| TEXAS INSTRUMENTS INCORPORATED
| Standard Linear and Logic Group
| IBIS Model of LVTH16245A
| 16-Bit Bus Transceiver with 3-State Outputs
| This file contains package information for the following:
|  SSOP 48-pin (DL) package as [Component] LVTH16245A_DL
|  TSSOP 48-pin (DGG) package as [Component] LVTH16245A_DGG
|  TVSOP 48-pin (DGV) package as [Component] LVTH16245A_DGV
|  jrBGA 48-pin (GQL) package as [Component] LVTH16245A_GQL
| This device can be powered at the following Vccs:
|  3.3 volt Vcc
|  2.7 volt Vcc
| This file provides unique models under the [Model Selector] for each Vcc.
| For operation at a specific Vcc, select the appropriate model after each
| [Model Selector] keyword.
[IBIS Ver]   3.2
[Comment char]  |_char
[File Name]   sn54lvth16245awd.ibs
[File Rev]   1.1 | g_die
[Date]   October 15, 2008
[Source]   Data created from TI-SPICE simulations at TI-SLL.
[Notes]   The following is an IBIS list for the LVTH16245A.
   Please contact sllibis@ti.com with questions and
   comments concerning SLL IBIS models.
   - FILE REV HISTORY
   - 1.1 Release IBIS file on 10/15/08
   - Power-clamp data has been deleted since there is no
   power-clamp diode in the device.
   - Due to presence of bus hold at input, GND-clamp curves
   have non-monotonic warnings.
   - Due to the fact that the device is 5-V input/output
   tolerant, the pullup and pulldown data has some
   non-monotonic warnings.
|08/13/2013  - Updated with ceramic 48WD parasitics.  WVB
[Disclaimer] Property of Texas Instruments Incorporated.  Unauthorized
   reproduction and/or distribution is strictly prohibited.
   This product is protected under copyright law.
   Created  2008, (C) Copyright  2008, Texas Instruments
   Incorporated, All Rights Reserved
   UNLESS THERE IS A SIGNED, WRITTEN AGREEMENT TO THE
   CONTRARY, TEXAS INSTRUMENTS (TI) IS PROVIDING THE IBIS
   MODELS  AND WITHOUT ANY WARRANTY, EXPRESSED OR
   IMPLIED.  TI assumes no liability for:
   1) the accuracy of the IBIS models provided to your
   company;
   2) the proper functioning of these IBIS Models in your
   design or for any resulting applications; or
   3) infringement of patents, copyrights or intellectual
   property rights resulting from your use of these IBIS
   models.
   TI provides IBIS Models as a service to our customers.
   You and your company shall not distribute, sell or give
   these models to anyone else without prior written
   permission from TI.
   TI reserves the right to make changes to our products or
   to discontinue any semiconductor product or service
   without notice, and advises our customers to obtain the
   latest version of relevant information to verify, before
   placing orders, that the information being relied on is
   current.
   Please be aware that your receipt and use of the IBIS
   information provided shall serve as acceptance of these
   terms and conditions.  If you do not accept these terms,
   you should return or destroy the IBIS models and any
   other accompanying information immediately.
|   48-pin ceramic (WD) packageP
[Component]   LVTH16245A_DL
[Manufacturer]   Texas Instruments, Inc.
[Package]
|   typ   min   max
R_pkg   0.161   0.116   0.231
L_pkg   6.816e-9   4.867e-9   10.108e-9
C_pkg   2.468e-12   1.62e-12   3.698e-12
[Pin]   signal_name   model_name   R_pin   L_pin   C_pin
1   S1DIR   LVTH16245E_IN   0.231   10.108e-9   3.220e-12
2   S1B1   LVTH16245E_IO   0.224   9.570e-9   3.698e-12
3   S1B2   LVTH16245E_IO   0.202   8.681e-9   3.350e-12
4   GND   GND   0.185   7.877e-9   2.960e-12
5   S1B3   LVTH16245E_IO   0.170   7.118e-9   2.404e-12
6   S1B4   LVTH16245E_IO   0.155   6.481e-9   2.131e-12
7   VCC   POWER   0.138   5.760e-9   2.150e-12
8   S1B5   LVTH16245E_IO   0.135   5.641e-9   2.103e-12
9   S1B6   LVTH16245E_IO   0.134   5.593e-9   2.070e-12
10   GND   GND   0.120   5.070e-9   1.812e-12
11   S1B7   LVTH16245E_IO   0.119   5.022e-9   1.793e-12
12   S1B8   LVTH16245E_IO   0.116   4.868e-9   1.651e-12
13   S2B1   LVTH16245E_IO   0.116   4.867e-9   1.658e-12
14   S2B2   LVTH16245E_IO   0.119   5.024e-9   1.805e-12
15   GND   GND   0.121   5.074e-9   1.825e-12
16   S2B3   LVTH16245E_IO   0.134   5.595e-9   2.105e-12
17   S2B4   LVTH16245E_IO   0.136   5.644e-9   2.144e-12
18   VCC   POWER   0.139   5.763e-9   2.197e-12
19   S2B5   LVTH16245E_IO   0.155   6.483e-9   2.152e-12
20   S2B6   LVTH16245E_IO   0.157   6.535e-9   2.172e-12
21   GND   GND   0.164   6.944e-9   2.459e-12
22   S2B7   LVTH16245E_IO   0.174   7.397e-9   2.657e-12
23   S2B8   LVTH16245E_IO   0.189   7.964e-9   2.834e-12
24   S2DIR   LVTH16245E_IN   0.188   8.149e-9   2.455e-12
25   S2NOE   LVTH16245E_IN   0.188   8.148e-9   2.455e-12
26   S2A8   LVTH16245E_IO   0.189   7.963e-9   2.834e-12
27   S2A7   LVTH16245E_IO   0.174   7.396e-9   2.658e-12
28   GND   GND   0.164   6.943e-9   2.461e-12
29   S2A6   LVTH16245E_IO   0.157   6.535e-9   2.174e-12
30   S2A5   LVTH16245E_IO   0.168   7.064e-9   2.384e-12
31   VCC   POWER   0.159   6.694e-9   2.687e-12
32   S2A4   LVTH16245E_IO   0.163   6.925e-9   2.828e-12
33   S2A3   LVTH16245E_IO   0.169   7.198e-9   2.967e-12
34   GND   GND   0.163   7.027e-9   2.887e-12
35   S2A2   LVTH16245E_IO   0.162   6.977e-9   2.868e-12
36   S2A1   LVTH16245E_IO   0.167   7.207e-9   2.815e-12
37   S1A8   LVTH16245E_IO   0.149   6.371e-9   2.557e-12
38   S1A7   LVTH16245E_IO   0.139   5.942e-9   2.312e-12
39   GND   GND   0.149   6.375e-9   2.428e-12
40   S1A6   LVTH16245E_IO   0.135   5.649e-9   2.135e-12
41   S1A5   LVTH16245E_IO   0.137   5.708e-9   2.174e-12
42   VCC   POWER   0.129   5.341e-9   1.804e-12
43   S1A4   LVTH16245E_IO   0.124   5.115e-9   1.620e-12
44   S1A3   LVTH16245E_IO   0.170   7.117e-9   2.402e-12
45   GND   GND   0.185   7.876e-9   2.956e-12
46   S1A2   LVTH16245E_IO   0.202   8.680e-9   3.347e-12
47   S1A1   LVTH16245E_IO   0.224   9.570e-9   3.696e-12
48   S1NOE   LVTH16245E_IN   0.231   10.108e-9   3.219e-12
| Component LVTH16245A_DGG 48-PIN TSSOP
[Component]   LVTH16245A_DGG
[Manufacturer]   Texas Instruments, Inc.
[Package]
|   typ   min   max
R_pkg   4.400e-02   3.800e-02   5.100e-02
L_pkg   3.019e-09   2.486e-09   4.099e-09
C_pkg   5.070e-13   3.340e-13   8.090e-13
[Pin]   signal_name   model_name   R_pin   L_pin   C_pin
1   S1DIR   LVTH16245E_IN   4.100e-02   4.017e-09   7.590e-13
2   S1B1   LVTH16245E_IO   4.200e-02   3.737e-09   7.920e-13
3   S1B2   LVTH16245E_IO   4.200e-02   3.480e-09   6.610e-13
4   GND   GND   3.800e-02   3.131e-09   5.750e-13
5   S1B3   LVTH16245E_IO   4.700e-02   3.122e-09   5.660e-13
6   S1B4   LVTH16245E_IO   4.300e-02   2.948e-09   5.040e-13
7   VCC   POWER   4.500e-02   2.845e-09   3.970e-13
8   S1B5   LVTH16245E_IO   4.900e-02   2.835e-09   3.940e-13
9   S1B6   LVTH16245E_IO   4.800e-02   2.715e-09   3.780e-13
10   GND   GND   5.000e-02   2.664e-09   3.630e-13
11   S1B7   LVTH16245E_IO   5.000e-02   2.585e-09   3.480e-13
12   S1B8   LVTH16245E_IO   4.900e-02   2.550e-09   3.370e-13
13   S2B1   LVTH16245E_IO   4.900e-02   2.541e-09   3.360e-13
14   S2B2   LVTH16245E_IO   5.000e-02   2.574e-09   3.480e-13
15   GND   GND   4.900e-02   2.618e-09   3.590e-13
16   S2B3   LVTH16245E_IO   4.600e-02   2.671e-09   3.750e-13
17   S2B4   LVTH16245E_IO   4.500e-02   2.754e-09   3.890e-13
18   VCC   POWER   4.400e-02   2.823e-09   4.500e-13
19   S2B5   LVTH16245E_IO   4.200e-02   2.968e-09   5.030e-13
20   S2B6   LVTH16245E_IO   5.100e-02   3.108e-09   5.350e-13
21   GND   GND   4.200e-02   3.175e-09   5.870e-13
22   S2B7   LVTH16245E_IO   4.100e-02   3.449e-09   6.780e-13
23   S2B8   LVTH16245E_IO   4.400e-02   3.766e-09   8.040e-13
24   S2DIR   LVTH16245E_IN   4.300e-02   4.065e-09   7.610e-13
25   S2NOE   LVTH16245E_IN   4.100e-02   3.994e-09   7.570e-13
26   S2A8   LVTH16245E_IO   3.900e-02   3.649e-09   7.890e-13
27   S2A7   LVTH16245E_IO   3.800e-02   3.362e-09   6.600e-13
28   GND   GND   3.800e-02   3.082e-09   5.740e-13
29   S2A6   LVTH16245E_IO   4.400e-02   2.990e-09   5.220e-13
30   S2A5   LVTH16245E_IO   4.100e-02   2.917e-09   4.950e-13
31   VCC   POWER   4.300e-02   2.820e-09   4.480e-13
32   S2A4   LVTH16245E_IO   4.300e-02   2.699e-09   3.850e-13
33   S2A3   LVTH16245E_IO   4.500e-02   2.628e-09   3.720e-13
34   GND   GND   4.600e-02   2.556e-09   3.560e-13
35   S2A2   LVTH16245E_IO   4.600e-02   2.495e-09   3.440e-13
36   S2A1   LVTH16245E_IO   4.700e-02   2.487e-09   3.340e-13
37   S1A8   LVTH16245E_IO   4.700e-02   2.490e-09   3.350e-13
38   S1A7   LVTH16245E_IO   4.600e-02   2.486e-09   3.430e-13
39   GND   GND   4.500e-02   2.566e-09   3.560e-13
40   S1A6   LVTH16245E_IO   4.400e-02   2.639e-09   3.740e-13
41   S1A5   LVTH16245E_IO   4.300e-02   2.701e-09   3.860e-13
42   VCC   POWER   4.300e-02   2.817e-09   4.500e-13
43   S1A4   LVTH16245E_IO   4.100e-02   2.935e-09   5.010e-13
44   S1A3   LVTH16245E_IO   4.700e-02   3.035e-09   5.290e-13
45   GND   GND   4.300e-02   3.171e-09   5.890e-13
46   S1A2   LVTH16245E_IO   4.000e-02   3.415e-09   6.820e-13
47   S1A1   LVTH16245E_IO   4.300e-02   3.741e-09   8.090e-13
48   S1NOE   LVTH16245E_IN   4.400e-02   4.099e-09   7.640e-13
| Component LVTH16245A_DGV 48-PIN TVSOP
[Component]   LVTH16245A_DGV
[Manufacturer]   Texas Instruments, Inc.
[Package]
|   typ   min   max
R_pkg   1.370e-01   1.010e-01   1.720e-01
L_pkg   3.632e-09   2.739e-09   5.243e-09
C_pkg   5.430e-13   4.100e-13   7.930e-13
[Pin]   signal_name   model_name   R_pin   L_pin   C_pin
1   S1DIR   LVTH16245E_IN   1.680e-01   5.238e-09   7.750e-13
2   S1B1   LVTH16245E_IO   1.660e-01   4.546e-09   6.740e-13
3   S1B2   LVTH16245E_IO   1.700e-01   4.356e-09   6.200e-13
4   GND   GND   1.720e-01   4.192e-09   5.310e-13
5   S1B3   LVTH16245E_IO   1.570e-01   3.821e-09   5.020e-13
6   S1B4   LVTH16245E_IO   1.430e-01   3.623e-09   5.600e-13
7   VCC   POWER   1.300e-01   3.292e-09   5.060e-13
8   S1B5   LVTH16245E_IO   1.190e-01   3.090e-09   4.520e-13
9   S1B6   LVTH16245E_IO   1.110e-01   2.927e-09   4.440e-13
10   GND   GND   1.050e-01   2.807e-09   4.350e-13
11   S1B7   LVTH16245E_IO   1.010e-01   2.739e-09   4.260e-13
12   S1B8   LVTH16245E_IO   1.020e-01   2.949e-09   5.040e-13
13   S2B1   LVTH16245E_IO   1.020e-01   2.960e-09   4.800e-13
14   S2B2   LVTH16245E_IO   1.010e-01   2.747e-09   4.100e-13
15   GND   GND   1.050e-01   2.809e-09   4.350e-13
16   S2B3   LVTH16245E_IO   1.110e-01   2.928e-09   4.440e-13
17   S2B4   LVTH16245E_IO   1.190e-01   3.090e-09   4.520e-13
18   VCC   POWER   1.300e-01   3.293e-09   5.120e-13
19   S2B5   LVTH16245E_IO   1.430e-01   3.622e-09   5.750e-13
20   S2B6   LVTH16245E_IO   1.570e-01   3.818e-09   5.200e-13
21   GND   GND   1.720e-01   4.186e-09   5.560e-13
22   S2B7   LVTH16245E_IO   1.700e-01   4.354e-09   6.430e-13
23   S2B8   LVTH16245E_IO   1.660e-01   4.544e-09   6.970e-13
24   S2DIR   LVTH16245E_IN   1.680e-01   5.240e-09   7.930e-13
25   S2NOE   LVTH16245E_IN   1.680e-01   5.243e-09   7.900e-13
26   S2A8   LVTH16245E_IO   1.660e-01   4.544e-09   6.940e-13
27   S2A7   LVTH16245E_IO   1.700e-01   4.351e-09   6.460e-13
28   GND   GND   1.720e-01   4.185e-09   5.630e-13
29   S2A6   LVTH16245E_IO   1.570e-01   3.817e-09   5.270e-13
30   S2A5   LVTH16245E_IO   1.430e-01   3.622e-09   5.790e-13
31   VCC   POWER   1.300e-01   3.293e-09   5.140e-13
32   S2A4   LVTH16245E_IO   1.190e-01   3.091e-09   4.560e-13
33   S2A3   LVTH16245E_IO   1.110e-01   2.928e-09   4.480e-13
34   GND   GND   1.050e-01   2.810e-09   4.380e-13
35   S2A2   LVTH16245E_IO   1.010e-01   2.748e-09   4.140e-13
36   S2A1   LVTH16245E_IO   1.020e-01   2.959e-09   4.830e-13
37   S1A8   LVTH16245E_IO   1.020e-01   2.949e-09   5.080e-13
38   S1A7   LVTH16245E_IO   1.010e-01   2.739e-09   4.300e-13
39   GND   GND   1.050e-01   2.806e-09   4.380e-13
40   S1A6   LVTH16245E_IO   1.110e-01   2.927e-09   4.480e-13
41   S1A5   LVTH16245E_IO   1.190e-01   3.091e-09   4.560e-13
42   VCC   POWER   1.300e-01   3.292e-09   5.110e-13
43   S1A4   LVTH16245E_IO   1.430e-01   3.623e-09   5.700e-13
44   S1A3   LVTH16245E_IO   1.570e-01   3.820e-09   5.150e-13
45   GND   GND   1.720e-01   4.189e-09   5.500e-13
46   S1A2   LVTH16245E_IO   1.700e-01   4.356e-09   6.370e-13
47   S1A1   LVTH16245E_IO   1.660e-01   4.547e-09   6.930e-13
48   S1NOE   LVTH16245E_IN   1.680e-01   5.233e-09   7.900e-13
| Component LVTH16245E_GQL 48-PIN JRBGA
[Component]   LVTH16245A_GQL
[Manufacturer]   Texas Instruments, Inc.
[Package]
|   typ   min   max
R_pkg   7.900e-02   4.500e-02   9.400e-02
L_pkg   2.264e-09   1.398e-09   2.722e-09
C_pkg   3.060e-13   1.170e-13   4.040e-13
[Pin]   signal_name   model_name   R_pin   L_pin   C_pin
A1   1DIR   LVTH16245E_DIR   5.100e-02   1.531e-09   2.100e-13
B2   1B1   LVTH16245E_IO   7.300e-02   2.572e-09   3.120e-13
B1   1B2   LVTH16245E_IO   7.100e-02   1.835e-09   2.320e-13
B3   GND   GND   9.400e-02   2.717e-09   3.830e-13
C2   1B3   LVTH16245E_IO   8.900e-02   2.534e-09   3.500e-13
C1   1B4   LVTH16245E_IO   7.100e-02   1.831e-09   2.310e-13
C3   VCC   POWER   9.400e-02   2.722e-09   3.920e-13
D2   1B5   LVTH16245E_IO   9.000e-02   2.551e-09   3.520e-13
D1   1B6   LVTH16245E_IO   7.200e-02   1.846e-09   2.440e-13
D3   GND   GND   9.400e-02   2.719e-09   4.030e-13
E2   1B7   LVTH16245E_IO   8.900e-02   2.541e-09   3.510e-13
E1   1B8   LVTH16245E_IO   7.200e-02   1.850e-09   2.270e-13
F1   2B1   LVTH16245E_IO   7.200e-02   1.850e-09   2.270e-13
F2   2B2   LVTH16245E_IO   8.900e-02   2.541e-09   3.510e-13
G3   GND   GND   9.400e-02   2.718e-09   4.040e-13
G1   2B3   LVTH16245E_IO   7.200e-02   1.847e-09   2.440e-13
G2   2B4   LVTH16245E_IO   9.000e-02   2.551e-09   3.520e-13
H3   VCC   POWER   9.400e-02   2.721e-09   3.920e-13
H1   2B5   LVTH16245E_IO   7.000e-02   1.830e-09   2.310e-13
H2   2B6   LVTH16245E_IO   8.800e-02   2.524e-09   3.500e-13
J3   GND   GND   9.300e-02   2.709e-09   3.820e-13
J1   2B7   LVTH16245E_IO   7.100e-02   1.851e-09   2.330e-13
J2   2B8   LVTH16245E_IO   5.600e-02   2.605e-09   3.900e-13
K1   2DIR   LVTH16245E_DIR   4.500e-02   1.398e-09   1.170e-13
K6   2NOE   LVTH16245E_NOE   4.500e-02   1.512e-09   1.930e-13
J5   2A8   LVTH16245E_IO   5.500e-02   2.492e-09   3.130e-13
J6   2A7   LVTH16245E_IO   7.000e-02   1.821e-09   2.300e-13
J4   GND   GND   9.300e-02   2.703e-09   3.820e-13
H5   2A6   LVTH16245E_IO   8.900e-02   2.529e-09   3.500e-13
H6   2A5   LVTH16245E_IO   7.100e-02   1.826e-09   2.300e-13
H4   VCC   POWER   9.400e-02   2.722e-09   3.910e-13
G5   2A4   LVTH16245E_IO   9.000e-02   2.551e-09   3.520e-13
G6   2A3   LVTH16245E_IO   7.200e-02   1.846e-09   2.440e-13
G4   GND   GND   9.400e-02   2.719e-09   4.040e-13
F5   2A2   LVTH16245E_IO   8.800e-02   2.510e-09   3.490e-13
F6   2A1   LVTH16245E_IO   7.200e-02   1.850e-09   2.270e-13
E6   1A8   LVTH16245E_IO   7.100e-02   1.850e-09   2.270e-13
E5   1A7   LVTH16245E_IO   8.900e-02   2.529e-09   3.500e-13
D4   GND   GND   9.400e-02   2.719e-09   4.030e-13
D6   1A6   LVTH16245E_IO   7.200e-02   1.847e-09   2.430e-13
D5   1A5   LVTH16245E_IO   8.900e-02   2.550e-09   3.520e-13
C4   VCC   POWER   9.400e-02   2.722e-09   3.910e-13
C6   1A4   LVTH16245E_IO   7.100e-02   1.827e-09   2.300e-13
C5   1A3   LVTH16245E_IO   8.900e-02   2.539e-09   3.500e-13
B4   GND   GND   9.300e-02   2.705e-09   3.820e-13
B6   1A2   LVTH16245E_IO   7.100e-02   1.831e-09   2.270e-13
B5   1A1   LVTH16245E_IO   7.300e-02   2.685e-09   3.800e-13
A6   1NOE   LVTH16245E_NOE   5.100e-02   1.417e-09   1.330e-13
| Model LVTH16245E_NOE
[Model Selector]   LVTH16245E_NOE
LVTH16245E_NOE_33   3.3 volt Vcc
LVTH16245E_NOE_27   2.7 volt Vcc
| Model LVTH16245E_DIR
[Model Selector]   LVTH16245E_DIR
LVTH16245E_DIR_33   3.3 volt Vcc
LVTH16245E_DIR_27   2.7 volt Vcc
| Model LVTH16245E_IN
[Model Selector]   LVTH16245E_IN
LVTH16245E_IN_33   3.3 volt Vcc
LVTH16245E_IN_27   2.7 volt Vcc
| Model LVTH16245E_IO
[Model Selector]   LVTH16245E_IO
LVTH16245E_IO_33   3.3 volt Vcc
LVTH16245E_IO_27   2.7 volt Vcc
| Models and submodels in the file (8): LVTH16245E_NOE_33 (Input), LVTH16245E_NOE_27 (Input), LVTH16245E_DIR_33 (Input), LVTH16245E_DIR_27 (Input), LVTH16245E_IN_33 (Input), LVTH16245E_IN_27 (Input), LVTH16245E_IO_33 (I/O), LVTH16245E_IO_27 (I/O)
